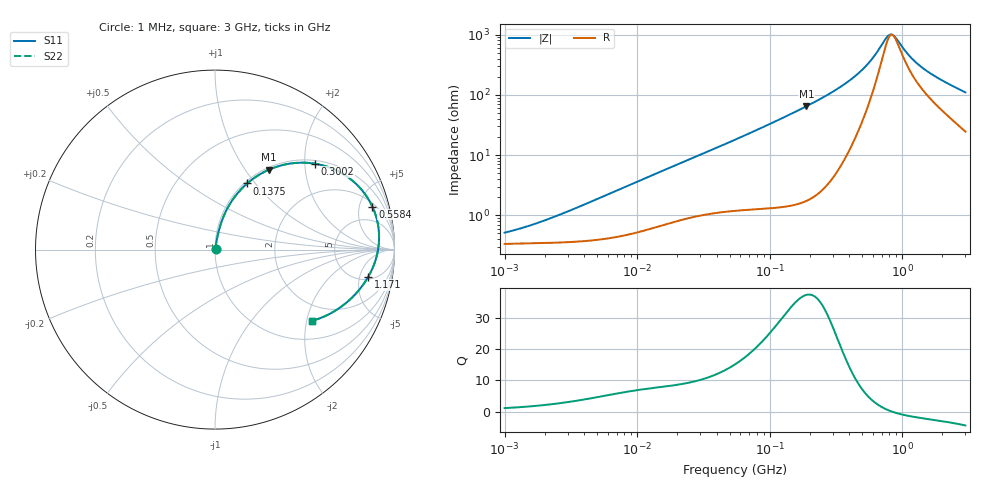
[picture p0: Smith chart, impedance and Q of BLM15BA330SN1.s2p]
! BLM15BA330SN1
# Hz S RI R 50
!Freq.(Hz) S11(Real) S11(Imag) S21(Real) S21(Imag) S12(Real) S12(Imag) S22(Real) S22(Imag)
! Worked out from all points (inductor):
!   401 points, 1 MHz to 3 GHz, reference 50 ohm
!   read as one part in series: L = 58.2 nH near 2.947 MHz
!   highest Q = 37.3 at 189.5 MHz (marker M1), where L = 54.2 nH
!   self-resonance near 844.2 MHz
!   S11 on the Smith chart (normalised r, x): 1 MHz: 1.01, +0.01; 137.5 MHz: 1.03, +0.91; 300.2 MHz: 1.08, +2.26; 558.4 MHz: 2.39, +6.60; 1.171 GHz: 5.58, -6.83; 3 GHz: 1.49, -2.15
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1000000  0.00334 0.00387  0.9967 -0.00387  0.9967 -0.00387  0.00334 0.00387
1786863  0.00346 0.00662  0.9965 -0.00662  0.9965 -0.00662  0.00346 0.00662
3823119  0.00387 0.0139  0.9961 -0.0139  0.9961 -0.0139  0.00387 0.0139
1.461624e7  0.00907 0.0504  0.9909 -0.0504  0.9909 -0.0504  0.00907 0.0504
3.00453e7  0.0195 0.0977  0.9805 -0.0977  0.9805 -0.0977  0.0195 0.0977
5.477226e7  0.0417 0.1695  0.9583 -0.1695  0.9583 -0.1695  0.0417 0.1695
9.216659e7  0.0927 0.2694  0.9073 -0.2694  0.9073 -0.2694  0.0927 0.2694
1.375402e8  0.1794 0.3685  0.8206 -0.3685  0.8206 -0.3685  0.1794 0.3685
1.894586e8  0.2993 0.4448  0.7007 -0.4448  0.7007 -0.4448  0.2993 0.4448
2.094008e8  0.3478 0.463  0.6522 -0.463  0.6522 -0.463  0.3478 0.463
3.002264e8  0.5586 0.4783  0.4414 -0.4783  0.4414 -0.4783  0.5586 0.4783
4.219165e8  0.7632 0.3862  0.2368 -0.3862  0.2368 -0.3862  0.7632 0.3862
5.583748e8  0.8768 0.2397  0.1232 -0.2397  0.1232 -0.2397  0.8768 0.2397
6.296259e8  0.902 0.1681  0.098 -0.1681  0.098 -0.1681  0.902 0.1681
7.539071e8  0.9142 0.0621  0.0858 -0.0621  0.0858 -0.0621  0.9142 0.0621
8.005644e8  0.9123 0.0285  0.0877 -0.0285  0.0877 -0.0285  0.9123 0.0285
8.332625e8  0.9097 0.00679  0.0903 -0.00679  0.0903 -0.00679  0.9097 0.00679
8.848309e8  0.9038 -0.0246  0.0962 0.0246  0.0962 0.0246  0.9038 -0.0246
1.171007e9  0.8536 -0.1518  0.1464 0.1518  0.1464 0.1518  0.8536 -0.1518
1.402151e9  0.8081 -0.2183  0.1919 0.2183  0.1919 0.2183  0.8081 -0.2183
1.712864e9  0.7491 -0.2809  0.2509 0.2809  0.2509 0.2809  0.7491 -0.2809
3e9  0.5392 -0.3971  0.4608 0.3971  0.4608 0.3971  0.5392 -0.3971
